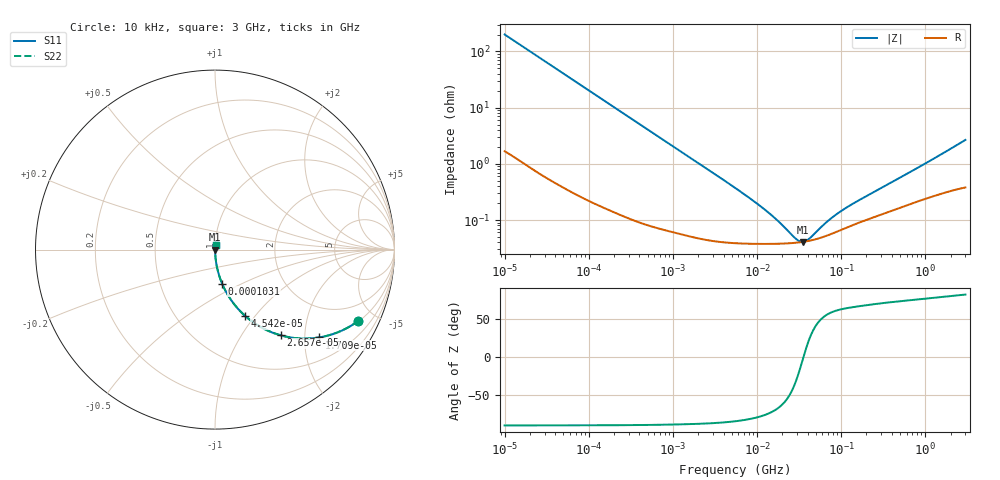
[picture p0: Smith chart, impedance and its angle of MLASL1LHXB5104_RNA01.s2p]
! MLASL1LHXB5104_RNA01  S-PARAMETER MODEL  ( Standard Model )
! Model Generated by TAIYO YUDEN Corporation (http://www.ty-top.com)
! Version 1.0
! TAIYO YUDEN Control No. 220601
! Copyright(c) 2015 TAIYO YUDEN CO.,LTD. All Rights Reserved.
! Product Description (link to TY-COMPAS)
! https://ds.yuden.co.jp/TYCOMPAS/or/detail?pn=MLASL1LHXB5104MRNA01&u=M
! Products Name : Multilayer Ceramic Capacitors
! Characteristics :
!  Capacitance : 0.1 [uF] , Rated Voltage : 10 [V] , TCC : X5R
!  Case Size : 1.0 x 0.5 / 0.039 x 0.02 [mm/inch] , Thickness : 0.13 / 0.005 [mm/inch]
!  (Conditions: Temperature = 25 [degC] , DC Bias Voltage = 0 [V])
! External Node Assignments :
!  1  o---| |---o  2
! GND o---------o GND
! Frequency Range : 10kHz  -  3GHz  [ 401 STEP ]
# MHZ S RI R 50
! Freq[MHz].  S11 Real  S11 Imag  S21 Real  S21 Imag  S12 Real  S12 Imag  S22 Real  S22 Imag
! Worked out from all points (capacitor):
!   401 points, 10 kHz to 3 GHz, reference 50 ohm
!   read as one part in series: C = 79.1 nF near 10.65 kHz
!   lowest |Z| = 40.8 mohm at 35.19 MHz (marker M1)
!   series resonance near 35.66 MHz, so ESL is about 250 pH
!   S11 on the Smith chart (normalised r, x): 10 kHz: 1.03, -4.02; 17.09 kHz: 1.02, -2.36; 26.57 kHz: 1.01, -1.52; 45.42 kHz: 1.01, -0.89; 103.1 kHz: 1.00, -0.39; 3 GHz: 1.01, +0.05
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0.01  0.7995 -0.3962  0.2005 0.3962  0.2005 0.3962  0.7995 -0.3962
0.01247  0.7208 -0.4444  0.2792 0.4444  0.2792 0.4444  0.7208 -0.4444
0.017091  0.5811 -0.4891  0.4189 0.4891  0.4189 0.4891  0.5811 -0.4891
0.026575  0.3674 -0.4778  0.6326 0.4778  0.6326 0.4778  0.3674 -0.4778
0.035295  0.2492 -0.4282  0.7508 0.4282  0.7508 0.4282  0.2492 -0.4282
0.045421  0.1682 -0.3695  0.8318 0.3695  0.8318 0.3695  0.1682 -0.3695
0.082683  0.059 -0.2306  0.941 0.2306  0.941 0.2306  0.059 -0.2306
0.103102  0.0394 -0.1891  0.9606 0.1891  0.9606 0.1891  0.0394 -0.1891
0.234035  0.00878 -0.0865  0.9912 0.0865  0.9912 0.0865  0.00878 -0.0865
0.683653  0.00161 -0.03  0.9984 0.03  0.9984 0.03  0.00161 -0.03
5.477226  0.0004 -0.00372  0.9996 0.00372  0.9996 0.00372  0.0004 -0.00372
14.10408  0.000377 -0.00125  0.9996 0.00125  0.9996 0.00125  0.000377 -0.00125
29.12589  0.000394 -0.000238  0.9996 0.000238  0.9996 0.000238  0.000394 -0.000238
32.0153  0.0004 -0.000126  0.9996 0.000126  0.9996 0.000126  0.0004 -0.000126
35.19136  0.000408 -1.53e-05  0.9996 1.53e-05  0.9996 1.53e-05  0.000408 -1.53e-05
39.92153  0.000421 0.000131  0.9996 -0.000131  0.9996 -0.000131  0.000421 0.000131
45.28751  0.000438 0.000278  0.9996 -0.000278  0.9996 -0.000278  0.000438 0.000278
66.11379  0.00052 0.000734  0.9995 -0.000734  0.9995 -0.000734  0.00052 0.000734
96.51742  0.000653 0.00123  0.9993 -0.00123  0.9993 -0.00123  0.000653 0.00123
150.0738  0.000858 0.00191  0.9991 -0.00191  0.9991 -0.00191  0.000858 0.00191
374.4521  0.00143 0.00423  0.9986 -0.00423  0.9986 -0.00423  0.00143 0.00423
3000  0.00447 0.0262  0.9955 -0.0262  0.9955 -0.0262  0.00447 0.0262
